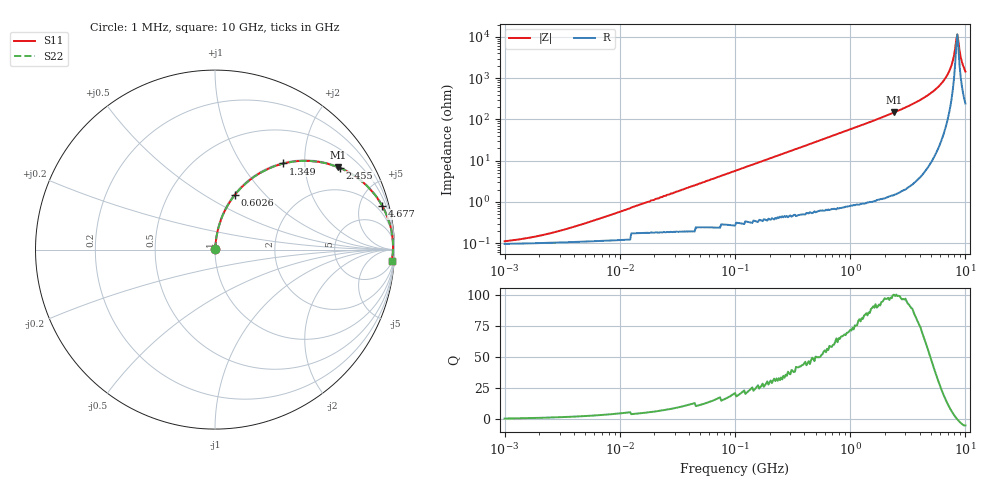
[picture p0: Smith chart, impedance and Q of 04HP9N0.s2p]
# MHz S MA R 50
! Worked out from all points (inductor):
!   401 points, 1 MHz to 10 GHz, reference 50 ohm
!   read as one part in series: L = 9 nH near 6.026 MHz
!   highest Q = 99.5 at 2.399 GHz (marker M1), where L = 9.78 nH
!   self-resonance near 8.318 GHz
!   S11 on the Smith chart (normalised r, x): 1 MHz: 1.00, +0.00; 602.6 MHz: 1.01, +0.68; 1.349 GHz: 1.02, +1.57; 2.455 GHz: 1.03, +3.03; 4.677 GHz: 1.13, +7.59; 10 GHz: 6, -29
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1  0.00108 31.5  0.999 -0.0  0.999 -0.0  0.00108 31.5
2.042  0.001536 48.6  0.999 -0.1  0.999 -0.1  0.001536 48.6
4.677  0.002892 65.8  0.999 -0.2  0.999 -0.2  0.002892 65.8
21.878  0.012 81.3  0.998 -0.7  0.998 -0.7  0.012 81.3
102.329  0.058 83.8  0.995 -3.3  0.995 -3.3  0.058 83.8
467.735  0.255 74.0  0.962 -14.8  0.962 -14.8  0.255 74.0
602.56  0.322 70.2  0.941 -18.8  0.941 -18.8  0.322 70.2
912.011  0.46 61.8  0.881 -27.4  0.881 -27.4  0.46 61.8
1348.963  0.613 51.5  0.783 -37.8  0.783 -37.8  0.613 51.5
2187.762  0.794 36.8  0.599 -52.6  0.599 -52.6  0.794 36.8
2398.833  0.824 34.0  0.559 -55.5  0.559 -55.5  0.824 34.0
2454.709  0.831 33.3  0.548 -56.2  0.548 -56.2  0.831 33.3
4677.351  0.963 14.7  0.254 -74.3  0.254 -74.3  0.963 14.7
5888.437  0.983 8.8  0.154 -79.2  0.154 -79.2  0.983 8.8
6918.31  0.99 4.9  0.086 -80.9  0.086 -80.9  0.99 4.9
7585.776  0.992 2.7  0.048 -78.6  0.048 -78.6  0.992 2.7
8128.305  0.992 1.1  0.02 -65.5  0.02 -65.5  0.992 1.1
8317.638  0.992 0.5  0.012 -46.7  0.012 -46.7  0.992 0.5
8511.38  0.991 -0.0  0.008639 3.3  0.008639 3.3  0.991 -0.0
8709.636  0.991 -0.6  0.013 47.5  0.013 47.5  0.991 -0.6
9549.926  0.988 -2.7  0.049 74.9  0.049 74.9  0.988 -2.7
10000  0.986 -3.8  0.068 76.5  0.068 76.5  0.986 -3.8
